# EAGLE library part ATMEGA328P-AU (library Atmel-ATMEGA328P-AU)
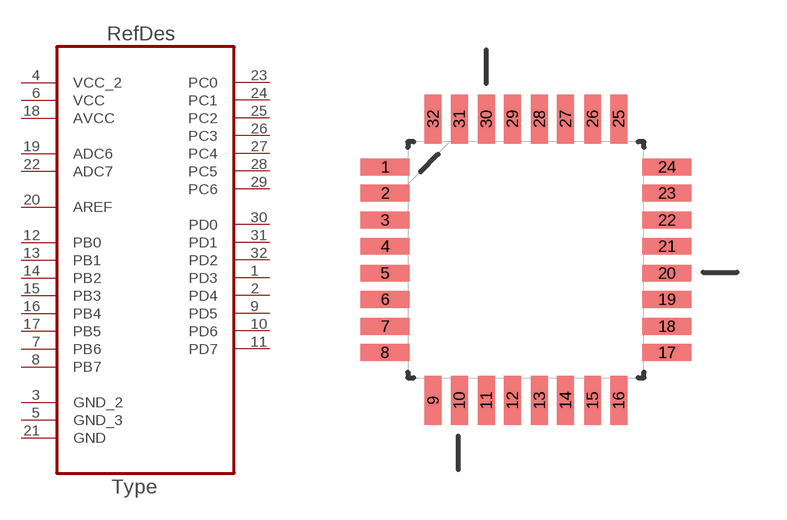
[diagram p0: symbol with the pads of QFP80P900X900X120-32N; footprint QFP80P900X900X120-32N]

Designator prefix U

## ATMEGA328P-AU (DESCRIPTION: 8-bit Microcontroller with In-System Programmable Flash; MPN: ATMEGA328P-AU; OC_FARNELL: 1715486; OC_NEWARK: 14R4631; PACKAGE: TQFP-32; SUPPLIER: Atmel)  [QFP80P900X900X120-32N]
1  PD3
2  PD4
3  GND_2  pas
4  VCC_2  pwr
5  GND_3  pas
6  VCC  pwr
7  PB6
8  PB7
9  PD5
10  PD6
11  PD7
12  PB0
13  PB1
14  PB2
15  PB3
16  PB4
17  PB5
18  AVCC  pwr
19  ADC6  in
20  AREF  in
21  GND  pas
22  ADC7  in
23  PC0
24  PC1
25  PC2
26  PC3
27  PC4
28  PC5
29  PC6
30  PD0
31  PD1
32  PD2

## Footprint QFP80P900X900X120-32N (pad centres in mm)
smd 1.473 x 0.508: 1 -4.242,2.794; 2 -4.242,2.007; 3 -4.242,1.194; 4 -4.242,0.406; 5 -4.242,-0.406; 6 -4.242,-1.194; 7 -4.242,-2.007; 8 -4.242,-2.794; 17 4.242,-2.794; 18 4.242,-2.007; 19 4.242,-1.194; 20 4.242,-0.406; 21 4.242,0.406; 22 4.242,1.194; 23 4.242,2.007; 24 4.242,2.794
smd 0.508 x 1.473: 9 -2.794,-4.242; 10 -2.007,-4.242; 11 -1.194,-4.242; 12 -0.406,-4.242; 13 0.406,-4.242; 14 1.194,-4.242; 15 2.007,-4.242; 16 2.794,-4.242; 25 2.794,4.242; 26 2.007,4.242; 27 1.194,4.242; 28 0.406,4.242; 29 -0.406,4.242; 30 -1.194,4.242; 31 -2.007,4.242; 32 -2.794,4.242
